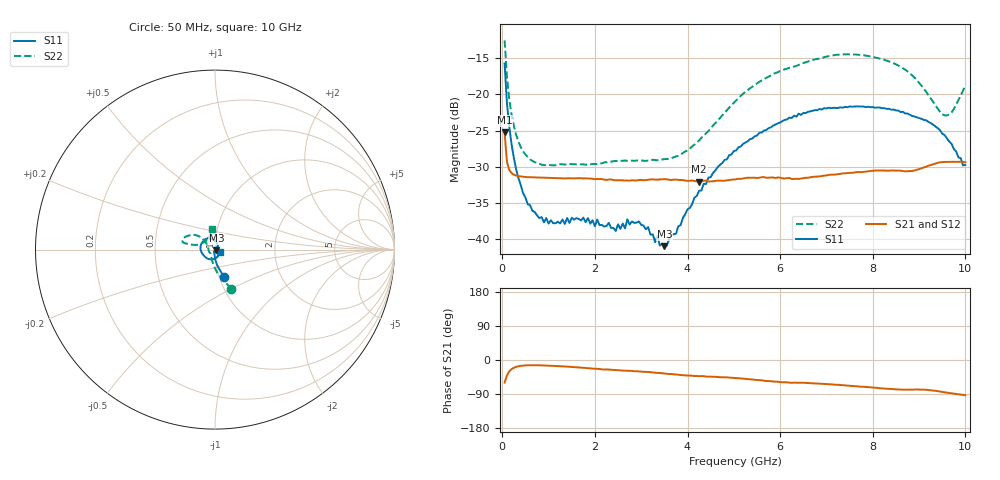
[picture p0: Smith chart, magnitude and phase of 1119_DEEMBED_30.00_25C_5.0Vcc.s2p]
!Hittite Microwave Corp.
!Digital Attenuator/PhaseShifter Rev 1.4.0
!Filename: C:\DATA\DATA\1119_DEEMBED_30.00_25C_5.0Vcc.s2p
!VNA ID: Agilent Technologies,N5224A,MY51441122,A.10.45.03
!Device type:
!2 Port Calibration.
!Temp(C): 25
!Lot Number:
!Serial Number:
!Operator:
!Misc:
!Attenuator:  30.000
# GHZ S DB R 50.0
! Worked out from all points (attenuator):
!   200 points, 50 MHz to 10 GHz, reference 50 ohm
!   highest |S21| = -25.26 dB at 50 MHz (marker M1); lowest = -32.0 dB at 4.25 GHz (marker M2)
!   lowest |S11| = -41.0 dB at 3.5 GHz (marker M3), VSWR 1.02, Z = 50.8 - j0.341 ohm
!   |S11| at or under -10 dB: start of sweep to end of sweep
!   |S22| runs from -29.8 to -12.6 dB; largest |S21 - S12| = 0.00011
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0.05  -15.75 -72.0  -25.26 -59.6  -25.26 -59.7  -12.56 -67.5
0.1  -21.17 -82.2  -29.30 -40.9  -29.28 -40.9  -17.51 -84.0
0.2  -26.89 -90.3  -30.87 -24.1  -30.88 -24.2  -22.78 -100.6
0.35  -31.60 -96.4  -31.29 -16.5  -31.29 -16.5  -26.56 -114.7
0.55  -35.19 -104.3  -31.43 -14.0  -31.43 -13.9  -28.66 -126.5
1  -37.84 -113.5  -31.53 -14.9  -31.53 -14.9  -29.74 -137.3
1.75  -37.02 -116.4  -31.61 -20.6  -31.60 -20.7  -29.67 -140.9
2.45  -38.87 -96.7  -31.85 -26.7  -31.85 -26.8  -29.18 -150.9
2.7  -37.26 -81.7  -31.89 -28.6  -31.90 -28.6  -29.18 -154.5
2.95  -37.55 -76.0  -31.82 -30.0  -31.83 -30.0  -29.15 -160.2
3.35  -39.55 -37.2  -31.79 -34.1  -31.78 -34.2  -29.11 -172.4
3.4  -40.86 -38.4  -31.74 -34.3  -31.75 -34.4  -29.05 -173.8
3.5  -40.96 -22.0  -31.70 -35.5  -31.69 -35.6  -28.94 -177.3
4.25  -33.30 44.1  -32.04 -42.6  -32.05 -42.7  -26.38 152.0
5.05  -27.74 78.1  -31.72 -47.6  -31.74 -47.6  -20.84 138.6
5.85  -24.32 105.7  -31.48 -56.9  -31.49 -56.9  -17.19 143.9
6.7  -22.28 129.8  -31.40 -61.5  -31.41 -61.4  -15.26 153.8
8.35  -21.99 -177.3  -30.54 -76.1  -30.54 -76.2  -15.45 168.1
8.9  -23.06 -150.9  -30.52 -77.9  -30.52 -77.8  -17.69 167.7
9.55  -25.62 -96.2  -29.33 -85.3  -29.35 -85.3  -22.90 138.1
9.7  -26.82 -79.9  -29.32 -87.8  -29.32 -87.8  -22.51 119.6
10  -29.74 -29.6  -29.38 -93.0  -29.38 -93.0  -18.76 98.2
